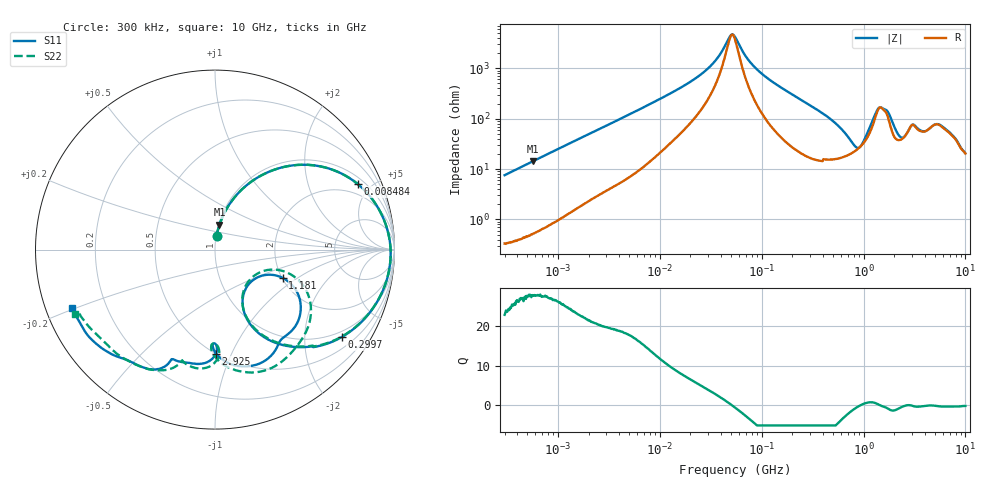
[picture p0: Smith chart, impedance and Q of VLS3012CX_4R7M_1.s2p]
! S-Parameter Data Generated by TDK Corporation
! Copyright(C) 2019 TDK Corporation.
! All Rights Reserved.
! TDK P/N: VLS3012CX-4R7M-1 (Inductor)
! Property: L=4.7uH at 1MHz
! Size(LxWxT): 3x3x1.2mm
! Model Type: s2p (Touchstone File Format Version 1.0)
! Frequency: DC=Yes Start=0.3MHz Stop=10000MHz 802points Log-sweep
! Model Generated on Sep. 23, 2019
! Port Assignments:
!  1 ---@@@--- 2
! Applicable Conditions:
!  Temperature = 25 degC
!  DC Bias Current = 0 A
!  Small Signal Operation
! Terms and conditions regarding TDK Simulation Models
! (1)This simulation model is being provided solely for informational purposes. Please refer to the specifications of the products in terms of detailed characteristics of such products.
! (2)In no event shall TDK Corporation of any of its subsidiaries be liable for any loss or damage arising, directly or indirectly,
!  From any information contained in this simulation model, including, but not limited to loss or damages arising from any inaccuracies, omissions or errors in connection with such information.
! (3)Any and all copyrights on this simulation model are owned by TDK Corporation.
!  Duplication or redistribution of this simulation model without prior written permission from TDK Corporation is prohibited.
! (4)This simulation model is subject to any modification or change without any prior notice.
! (5)Neither TDK Corporation nor any of its subsidiaries shall make any warranty, express or implied,
!  Including but not limited to the correctness, implied warranties of merchantability and fitness for a particular purpose with respect to this simulation models.
! (6)The use of this simulation model shall be deemed to have consented to the terms and conditions hereof.
# Hz S MA R 50
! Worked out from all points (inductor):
!   801 points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, 300 kHz to 10 GHz, reference 50 ohm
!   read as one part in series: L = 4 uH near 318.3 kHz
!   highest Q = 27.6 at 567.7 kHz (marker M1), where L = 4 uH
!   self-resonance near 51.43 MHz
!   S11 on the Smith chart (normalised r, x): 300 kHz: 1.01, +0.15; 8.484 MHz: 1.33, +4.15; 299.7 MHz: 0.82, -3.00; 1.181 GHz: 2.02, -0.77; 2.925 GHz: 0.50, -0.87; 10 GHz: 0.08, -0.20
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300000  0.07496 83.1  0.9939 -4.3  0.9939 -4.3  0.07477 83.2
567737  0.1403 79.8  0.985 -8.1  0.9851 -8.1  0.1401 79.8
1713600  0.3835 64.9  0.9065 -22.6  0.9065 -22.6  0.3834 64.9
3956438  0.6738 44.6  0.7038 -42.4  0.7039 -42.4  0.6737 44.6
8484346  0.8746 24.7  0.4234 -60.9  0.4234 -60.9  0.8746 24.8
9671944  0.895 21.9  0.3779 -63.4  0.3779 -63.4  0.895 21.9
2.630692e7  0.9681 6.0  0.1207 -72.1  0.1207 -72.1  0.9681 6.1
4.929468e7  0.979 -1.0  0.02218 -19.8  0.02219 -19.8  0.979 -0.9
5.477226e7  0.9793 -2.1  0.02321 25.2  0.02323 25.2  0.9793 -2.1
1.050124e8  0.9709 -10.5  0.1334 70.8  0.1334 70.8  0.9709 -10.3
2.996953e8  0.8573 -34.7  0.4456 50.5  0.4456 50.5  0.8573 -34.3
3.126428e8  0.8469 -36.1  0.4623 49.0  0.4623 49.0  0.8469 -35.7
5.046115e8  0.6619 -53.9  0.6513 27.5  0.6513 27.5  0.6619 -53.4
7.612374e8  0.3994 -65.3  0.7667 1.1  0.7666 1.1  0.3968 -65.0
9.789263e8  0.2689 -43.6  0.7464 -20.5  0.7465 -20.5  0.2569 -42.3
1.180962e9  0.4092 -22.7  0.6009 -39.8  0.6013 -39.8  0.4014 -17.5
1.403063e9  0.6094 -40.3  0.3585 -39.5  0.3593 -39.7  0.6447 -34.1
1.767019e9  0.674 -63.7  0.3817 -12.4  0.3804 -12.3  0.7299 -66.4
2.203374e9  0.5992 -87.8  0.5603 -25.8  0.5607 -25.7  0.5952 -90.1
2.924554e9  0.5819 -89.6  0.4379 -54.6  0.4381 -54.6  0.588 -87.8
5.76861e9  0.766 -120.4  0.2701 -74.9  0.2701 -74.8  0.7601 -118.7
1e10  0.8591 -157.8  0.1908 -96.1  0.1907 -96.3  0.8561 -155.4
